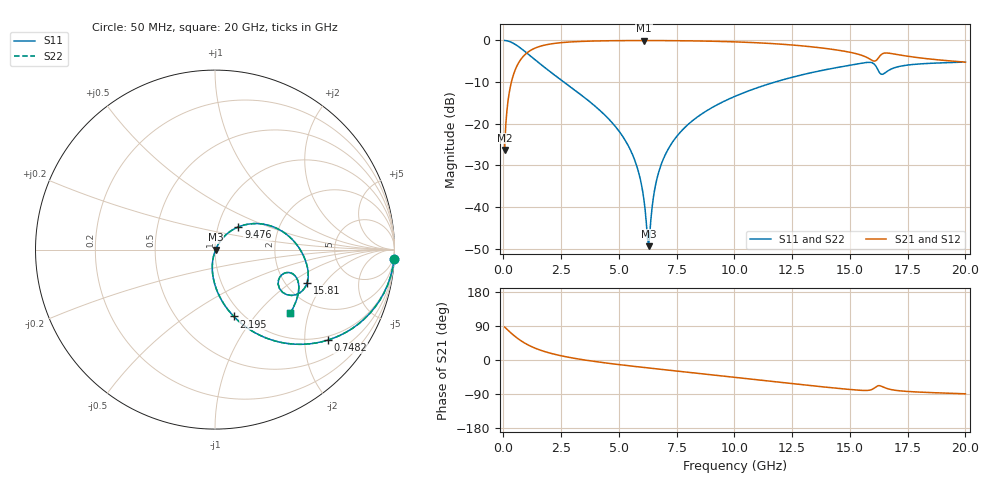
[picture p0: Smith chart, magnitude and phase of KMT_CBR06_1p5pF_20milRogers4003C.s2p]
! Data measured by Modelithics Inc. support@modelithics.com 813-866-6335
! KEMET CBR0603 1.5pF, Pad Width= 0.851mm, Pad Length= 0.64mm, Pad Gap= 0.62mm, 20mil Rogers 4003C substrate Data, January 2022
# hz S ma R 50
! 2 Port Network Data from SP1.SP block
! freq  magS11  angS11  magS21  angS21  magS12  angS12  magS22  angS22
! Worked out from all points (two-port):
!   401 points, 50 MHz to 20 GHz, reference 50 ohm
!   highest |S21| = -0.03 dB at 6.085 GHz (marker M1); lowest = -26.3 dB at 50 MHz (marker M2)
!   |S21| within 3 dB of the highest: 1.01 GHz to 15.16 GHz (14.15 GHz wide, 175 % of centre); 16.52 GHz to 16.63 GHz (118 MHz wide, 0.712 % of centre)
!   lowest |S11| = -49.4 dB at 6.284 GHz (marker M3), VSWR 1.01, Z = 50.3 - j0.0913 ohm
!   |S11| at or under -10 dB: 2.617 GHz to 11.76 GHz (9.138 GHz wide, 127 % of centre)
!   |S22| runs from -49.4 to 0.0 dB; largest |S21 - S12| = 0
!   S11 on the Smith chart (normalised r, x): 50 MHz: 1, -39; 748.2 MHz: 0.89, -2.57; 2.195 GHz: 0.90, -0.79; 9.476 GHz: 1.25, +0.33; 15.81 GHz: 2.59, -1.37; 20 GHz: 1.51, -1.54
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5e7  0.9988 -2.9  0.04827 87.1  0.04827 87.1  0.9988 -2.9
2.99375e8  0.9602 -17.2  0.2784 72.8  0.2784 72.8  0.9602 -17.2
7.4825e8  0.8062 -38.7  0.5903 51.2  0.5903 51.2  0.8062 -38.7
1.396625e9  0.5774 -59.3  0.8146 30.6  0.8146 30.6  0.5774 -59.3
2.194625e9  0.3868 -74.3  0.9199 15.4  0.9199 15.4  0.3868 -74.3
3.391625e9  0.2184 -88.2  0.9734 1.2  0.9734 1.2  0.2184 -88.2
5.286875e9  0.06213 -101.7  0.9951 -14.2  0.9951 -14.2  0.06213 -101.7
5.785625e9  0.03013 -102.0  0.9963 -17.7  0.9963 -17.7  0.03013 -102.0
6.084875e9  0.01206 -94.3  0.9965 -19.7  0.9965 -19.7  0.01206 -94.3
6.184625e9  0.006514 -80.1  0.9965 -20.4  0.9965 -20.4  0.006514 -80.1
6.284375e9  0.003388 -15.5  0.9964 -21.1  0.9964 -21.1  0.003388 -15.5
6.53375e9  0.01544 53.7  0.996 -22.8  0.996 -22.8  0.01544 53.7
6.73325e9  0.02686 57.7  0.9956 -24.1  0.9956 -24.1  0.02686 57.7
7.13225e9  0.04957 58.2  0.9941 -26.7  0.9941 -26.7  0.04957 58.2
7.680875e9  0.08043 55.9  0.9911 -30.3  0.9911 -30.3  0.08043 55.9
9.476375e9  0.1816 44.1  0.9708 -42.0  0.9708 -42.0  0.1816 44.1
1.0025e10  0.2133 40.1  0.9606 -45.6  0.9606 -45.6  0.2133 40.1
1.336662e10  0.4121 11.3  0.8366 -67.9  0.8366 -67.9  0.4121 11.3
1.58105e10  0.5456 -19.9  0.6084 -80.0  0.6084 -80.0  0.5456 -19.9
1.630925e10  0.4015 -28.7  0.6558 -68.0  0.6558 -68.0  0.4015 -28.7
1.670825e10  0.4416 -17.1  0.7019 -77.0  0.7019 -77.0  0.4416 -17.1
2e10  0.55 -40.2  0.5484 -89.2  0.5484 -89.2  0.55 -40.2
